(* Logix 5000 AddOnInstructionDefinition export Banner_ZMX_Control; software revision 33.03 *)

TYPE Banner_ZMX_Data :
STRUCT
   Data_In : Banner_ZMX_Data_In;
   Data_Out : Banner_ZMX_Data_Out;
   Unevenness : INT;
END_STRUCT
END_TYPE

TYPE Banner_ZMX_Data_In :
STRUCT
   Input_Ack : INT;
   Reserved1 : INT;
   Sensor_Fault_Code : INT;
   Boot_Count : INT;   // 1 to 65535
   Up_Time : DINT;   // 1 to 4294967295 in ms
   Missed_Trigger_Count : DINT;
   Reserved2 : INT;
   Reserved3 : INT;
   Reserved4 : INT;
   Reserved5 : INT;
   Reserved6 : INT;
   Reserved7 : INT;
   Reserved8 : INT;
   Reserved30 : INT;
   Frame_Number : DINT;
   Invalid_Pixel_Count : DINT;   // 0 to 56576. Pixels with too little light received to be able to measure.
   Saturated_Pixel_Count : DINT;   // 0 to 56576. Pixels with too much light received to be able to measure.
   Conf_Error_Code : INT;
   Reserved9 : INT;
   Fill_Level_Percent : INT;   // 0 to 200
   Peak_Height : INT;   // 0 to 3500 in mm
   Estimated_Item_Count : INT;
   Output_1_PFM : INT;   // 0. 100 to 600 Hz.
   Output_2_PFM : INT;   // 0. 100 to 600 Hz.
   Trigger_Mode : INT;   // 1 = External, 5 = Internal (uses trigger period), 6 = Free run, 10 = Softa
   Trigger_Period : INT;   // 200 to 60000 ms
   Illumination_Power_Percent : INT;   // 1 to 100
   Reserved10 : INT;
   Reserved11 : INT;
   Reserved12 : INT;
   Reserved13 : INT;
   Reserved14 : INT;
   Reserved15 : INT;
   Reserved16 : INT;
   Reserved17 : INT;
   Pitch_Angle : INT;   // -4500 to 4500 (degrees x 100)
   Roll_Angle : INT;   // -4500 to 4500 (degrees x 100)
   Yaw_Angle : INT;   // -18000 to 18000 (degrees x 100)
   Reserved18 : INT;
   Reserved19 : INT;
   Reserved20 : INT;
   Reserved31 : INT;
   Discrete_IO_Polarity : INT;   // 0 = PNP, 1 = NPN, 2 = Push-Pull
   Reserved21 : INT;
   Fill_Level_Limit_Setpoint_Percent : INT;   // 0 to 200 in mm
   Reserved22 : INT;
   Peak_Height_Limit_Setpoint : INT;   // 0 to 2950 mm
   Reserved23 : INT;
   Discrete_Output_1_Control_Mode : INT;   // 0 = Disabled, 1 = Fill % above setpoint, 2 = Peak height aboe setpoint, 9 = Fill % above setpoint or peak height above setpoint, 10 = Pulse Pro 100 to 600 Hz scaled between 0 to 100%, 11 = Pulse Pro 100 to 600 Hz scaled to peak height above bottom of container, 20 = No output, channle used as input.
   Discrete_Output_2_Control_Mode : INT;   // 0 = Disabled, 1 = Fill % above setpoint, 2 = Peak height aboe setpoint, 9 = Fill % above setpoint or peak height above setpoint, 10 = Pulse Pro 100 to 600 Hz scaled between 0 to 100%, 11 = Pulse Pro 100 to 600 Hz scaled to peak height above bottom of container, 20 = No output, channle used as input.
   ROI_Anchor_Point_X : INT;   // -2500 to 2500
   ROI_Anchor_Point_Y : INT;   // -2500 to 2500
   ROI_Anchor_Point_Z : INT;   // 200 to 3000
   ROI_Length_X : INT;   // 50 to 5000
   ROI_Width_Y : INT;   // 50 to 5000
   ROI_Height_Z : INT;   // 50 to 3000
   Reserved24 : INT;
END_STRUCT
END_TYPE

TYPE Banner_ZMX_Data_Out :
STRUCT
   Control_Bits : INT;
   Reserved1 : INT;
   Trigger_Mode : INT;   // 1 = External, 5 = Internal (uses trigger perdio), 6 = Free Run, 10 = Software
   Trigger_Period : INT;   // 100 to 60000 ms
   Illumination_Power_Precent : INT;   // 0 to 100
   Reserved2 : INT;
   Reserved3 : INT;
   Reserved4 : INT;
   Reserved5 : INT;
   Reserved6 : INT;
   Reserved7 : INT;
   Reserved8 : INT;
   Pitch_Angle : INT;   // -4500 to 4500 (degrees x 100)
   Roll_Angle : INT;   // -4500 to 4500 (degrees x 100)
   Yaw_Angle : INT;   // -18000 to 18000 (degrees x 100)
   Reserved9 : INT;
   Reserved10 : INT;
   Reserved11 : INT;
   Discrete_IO_Polarity : INT;   // 0 = PNP, 1 = NPN, 2 = Push Pull
   Reserved12 : INT;
   Fill_Level_Limit_Setpoint_Percent : INT;   // 0 to 200
   Reserved13 : INT;
   Peak_Height_Limit_Setpoint : INT;   // 0 to 2950 in mm
   Reserved14 : INT;
   Discrete_Output_1_Control_Mode : INT;   // 0 = Disabled, 1 = Fill % above setpoint, 2 = Peak height aboe setpoint, 9 = Fill % above setpoint or peak height above setpoint, 10 = Pulse Pro 100 to 600 Hz scaled between 0 to 100%, 11 = Pulse Pro 100 to 600 Hz scaled to peak height above bottom of container, 20 = No output, channle used as input.
   Discrete_Output_2_Control_Mode : INT;   // 0 = Disabled, 1 = Fill % above setpoint, 2 = Peak height aboe setpoint, 9 = Fill % above setpoint or peak height above setpoint, 10 = Pulse Pro 100 to 600 Hz scaled between 0 to 100%, 11 = Pulse Pro 100 to 600 Hz scaled to peak height above bottom of container, 20 = No output, channle used as input.
   ROI_Anchor_Point_X : INT;   // -2500 to 2500 in mm
   ROI_Anchor_Point_Y : INT;   // -2500 to 2500 in mm
   ROI_Anchor_Point_Z : INT;   // 200 to 3000 in mm
   ROI_Length_X : INT;   // 50 to 5000 in mm
   ROI_Width_Y : INT;   // 50 to 5000 in mm
   ROI_Height_Z : INT;   // 50 to 3000 in mm
   Reserved50 : INT[8];
END_STRUCT
END_TYPE

TYPE Banner_ZMX_Full_Recipe :   // Recipe Data elements. for a ZMX unit.
STRUCT
   Trigger_Mode : INT;   // 1 = External, 5 = Internal, 6 = Free Run, 10 = Software
   Trigger_Period : INT;   // 100 to 60000 in ms
   Illumination_Power : INT;   // 0 to 100
   Pitch_Angle : INT;   // -4500 to 4500
   Roll_Angle : INT;   // -4500 to 4500
   Yaw_Angle : INT;   // -18000 to 18000
   Discrete_IO_Polarity : INT;   // 0 = PNP, 1= NPN, 2 = Push Pull
   Fill_Level_Limit_Setpoint_Percent : INT;   // 0 to 200
   Reserved13 : INT;
   Peak_Height_Limit_Setpoint : INT;   // 0 to 2950 in mm
   Reserved14 : INT;
   Discrete_Output_1_Control_Mode : INT;   // 0 = Disabled, 1 = Fill % above setpoint, 2 = Peak height aboe setpoint, 9 = Fill % above setpoint or peak height above setpoint, 10 = Pulse Pro 100 to 600 Hz scaled between 0 to 100%, 11 = Pulse Pro 100 to 600 Hz scaled to peak height above bottom of container, 20 = No output, channle used as input.
   Discrete_Output_2_Control_Mode : INT;   // 0 = Disabled, 1 = Fill % above setpoint, 2 = Peak height aboe setpoint, 9 = Fill % above setpoint or peak height above setpoint, 10 = Pulse Pro 100 to 600 Hz scaled between 0 to 100%, 11 = Pulse Pro 100 to 600 Hz scaled to peak height above bottom of container, 20 = No output, channle used as input.
   ROI_Anchor_X : INT;   // -2500 to 2500 in mm
   ROI_Anchor_Y : INT;   // -2500 to 2500 in mm
   ROI_Anchor_Z : INT;   // 200 to 3000 in mm
   ROI_Length_X : INT;   // 50 to 5000 in mm
   ROI_Length_Y : INT;   // 50 to 5000 in mm
   ROI_Length_Z : INT;   // 50 to 3000 in mm
END_STRUCT
END_TYPE

ADD_ON_INSTRUCTION Banner_ZMX_Control   (* revision 1.2 *)
// Revision note:
// Cyclic operation timing adjusted. Now waits 600 msecs instead of 300 after Cyclic Bit is turned on. Also the error timer is now 5 seconds instead of 3.
VAR_IN_OUT
   BinFill_Update : BOOL; {required}
   Cyclic_Update : BOOL; {required}
   ZMX_Raw_Inputs : INT[68]; {required}
   ZMX_Raw_Outputs : INT[40]; {required}
END_VAR
VAR_INPUT
   ZMX_Status : BOOL; {required}
END_VAR
VAR_IN_OUT
   ZMX : Banner_ZMX_Data; {required}
   Parameter_Update : Banner_ZMX_Full_Recipe; {required}
        .TRIGGER_MODE   // Check Data 1
        .PEAK_HEIGHT_LIMIT_SETPOINT   // Check Data 2
        .DISCRETE_OUTPUT_1_CONTROL_MODE   // Check Data 3
        .DISCRETE_OUTPUT_2_CONTROL_MODE   // Check Data 4
        .ROI_ANCHOR_X   // Check Data 5
        .ROI_ANCHOR_Y   // Check Data 6
        .ROI_ANCHOR_Z   // Check Data 7
        .ROI_LENGTH_X   // Check Data 8
        .ROI_LENGTH_Y   // Check Data 9
        .ROI_LENGTH_Z   // Check Data 10
END_VAR
VAR_OUTPUT
   Busy : BOOL; {visible}
   Done : BOOL; {visible}
   Bin_Error : BOOL; {access Read Only, visible}
   Cyclic_Error : BOOL; {visible}
   Comms_Error : BOOL; {visible}
   Sensor_Fault : INT; {access Read Only, visible}
   Config_Error : INT; {access Read Only, visible}
END_VAR
VAR
   Local : DINT; {access None}
   InData : INT[70]; {access None}
   Timer1 : TIMER := (PRE := 3000); {access None}
   Timer2 : TIMER := (PRE := 5000); {access None}
   Value : DINT[2]; {access None}
END_VAR

ROUTINE Logic   (* ladder *)
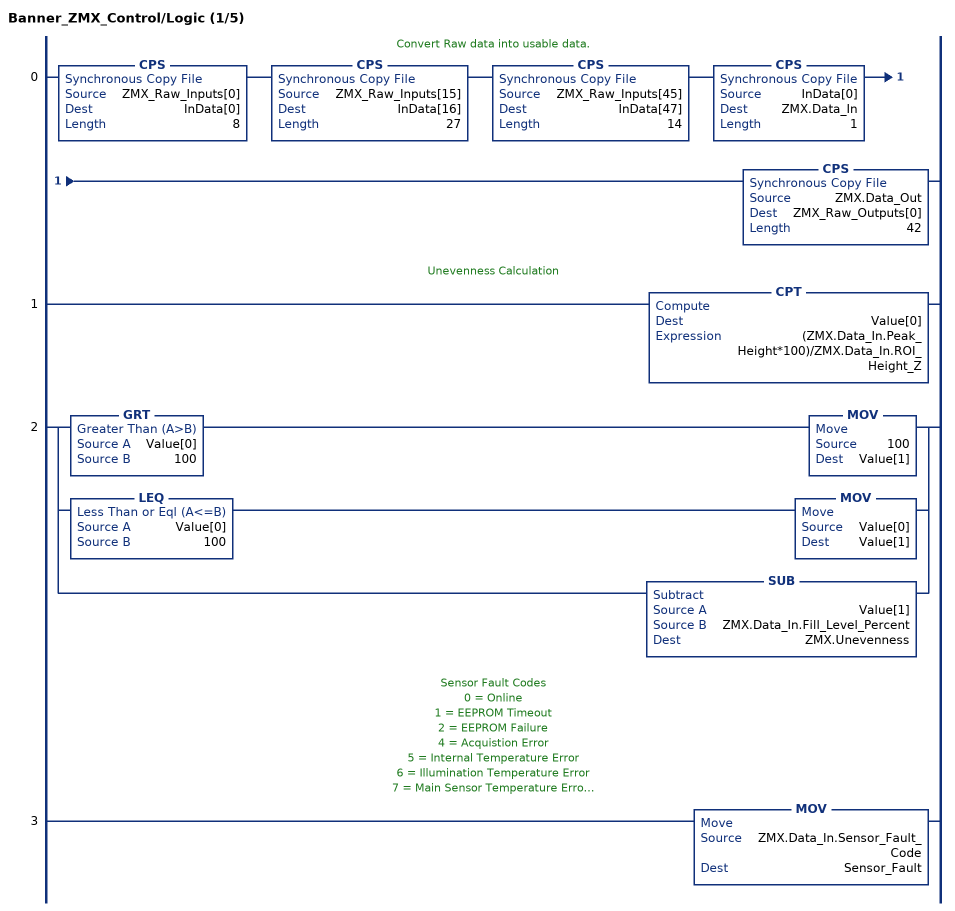
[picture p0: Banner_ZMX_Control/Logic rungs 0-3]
   // Convert Raw data into usable data.
   0: CPS(ZMX_Raw_Inputs[0],InData[0],8)CPS(ZMX_Raw_Inputs[15],InData[16],27)CPS(ZMX_Raw_Inputs[45],InData[47],14)CPS(InData[0],ZMX.Data_In,1)CPS(ZMX.Data_Out,ZMX_Raw_Outputs[0],42);
   // Unevenness Calculation
   1: CPT(Value[0],(ZMX.Data_In.Peak_Height*100)/ZMX.Data_In.ROI_Height_Z);
   2: [GRT(Value[0],100) MOV(100,Value[1]) ,LEQ(Value[0],100) MOV(Value[0],Value[1]) ,SUB(Value[1],ZMX.Data_In.Fill_Level_Percent,ZMX.Unevenness) ];
   // Sensor Fault Codes
   // 0 = Online
   // 1 = EEPROM Timeout
   // 2 = EEPROM Failure
   // 4 = Acquistion Error
   // 5 = Internal Temperature Error
   // 6 = Illumination Temperature Error
   // 7 = Main Sensor Temperature Error
   // 8 = Acquistion Error 2
   // 11 = Laser Operation Error
   // 20 = Internal Test Error
   // 21 = Internal Read Error
   // 22 = Internal Write Error
   // 30 = Laser Power Test Error
   // 31 = Laser Power Read Error
   // 32 = Laser Power Write Error
   // 1000 = Acquistion Error 3
   // 1011 to 1017 = Internal Flash Errors
   // 30000 to 32000 = Boot Loader Error
   3: MOV(ZMX.Data_In.Sensor_Fault_Code,Sensor_Fault);
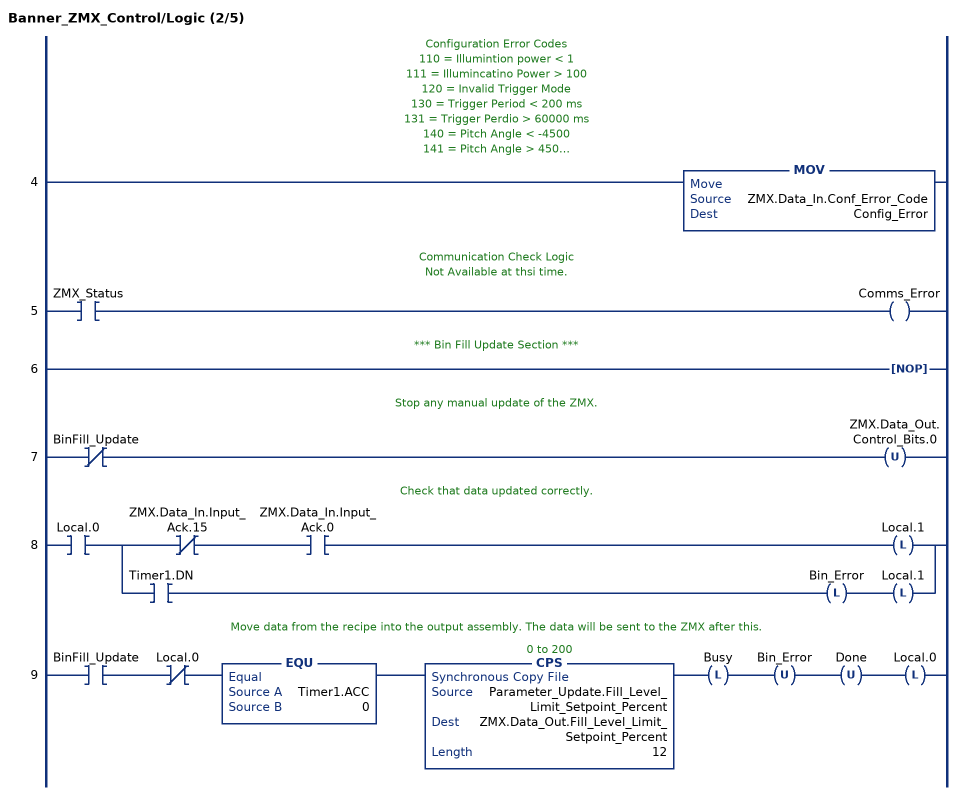
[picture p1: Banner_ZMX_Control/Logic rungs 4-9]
   // Configuration Error Codes
   // 110 = Illumintion power < 1
   // 111 = Illumincatino Power > 100
   // 120 = Invalid Trigger Mode
   // 130 = Trigger Period < 200 ms
   // 131 = Trigger Perdio > 60000 ms
   // 140 = Pitch Angle < -4500
   // 141 = Pitch Angle > 4500
   // 150 = Roll Angle < -4500
   // 151 = Roll Angle > 4500
   // 160 = Yaw Angle < -18000
   // 161 = Yaw Angle > 18000
   // 300 = Invalid Discrete Output
   // 2000 = Anchor Point X < -2500
   // 2001 = Anchor Point X > 2500
   // 2010 = Anchor Point Y < -2500
   // 2011 = Anchor Point Y > 2500
   // 2020 = Anchor Point Z < -2500
   // 2021 = Anchor Point Z > 2500
   // 2030 = Bin Length X < 50
   // 2031 = Bin Length X > 5000
   // 2040 = Bin Width < 50
   // 2041 = Bin Width > 5000
   // 2050 = Bin Width < 50
   // 2051 = Bin Width > 5000
   // 2052 = Invalid Bin Height
   // 2060 = Fill Level Setpoint < 0
   // 2061 = Fill Level Setpoint > 200
   // 2080 = Peak Height Setpoint < 0
   // 2081 = Peak Height Setpoint > Bin Height Z
   // 2100 = Discrete Out 1 Selection Invalid
   // 2110 = Discrete Out 2 Selectino Invalid
   4: MOV(ZMX.Data_In.Conf_Error_Code,Config_Error);
   // Communication Check Logic
   // Not Available at thsi time.
   5: XIC(ZMX_Status)OTE(Comms_Error);
   // *** Bin Fill Update Section ***
   6: NOP();
   // Stop any manual update of the ZMX.
   7: XIO(BinFill_Update)OTU(ZMX.Data_Out.Control_Bits.0);
   // Check that data updated correctly.
   8: XIC(Local.0)[XIO(ZMX.Data_In.Input_Ack.15) XIC(ZMX.Data_In.Input_Ack.0) OTL(Local.1) ,XIC(Timer1.DN) OTL(Bin_Error) OTL(Local.1) ];
   // Move data from the recipe into the output assembly. The data will be sent to the ZMX after this.
   9: XIC(BinFill_Update)XIO(Local.0)EQU(Timer1.ACC,0)CPS(Parameter_Update.Fill_Level_Limit_Setpoint_Percent,ZMX.Data_Out.Fill_Level_Limit_Setpoint_Percent,12)OTL(Busy)OTU(Bin_Error)OTU(Done)OTL(Local.0);
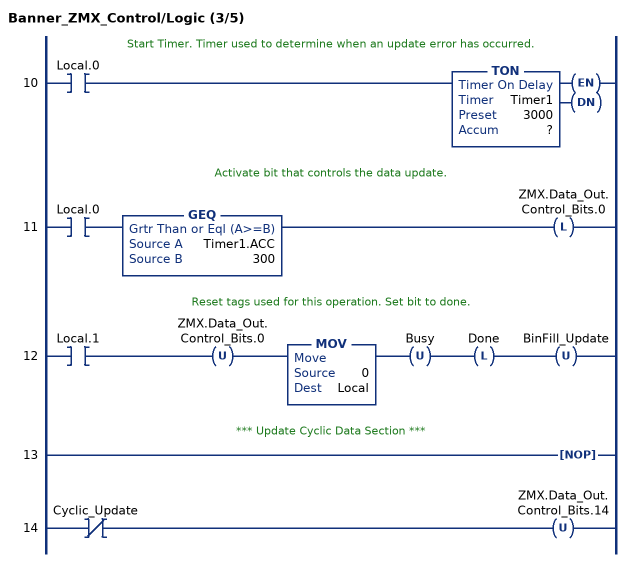
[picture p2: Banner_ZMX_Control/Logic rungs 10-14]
   // Start Timer. Timer used to determine when an update error has occurred.
   10: XIC(Local.0)TON(Timer1,?,?);
   // Activate bit that controls the data update.
   11: XIC(Local.0)GEQ(Timer1.ACC,300)OTL(ZMX.Data_Out.Control_Bits.0);
   // Reset tags used for this operation. Set bit to done.
   12: XIC(Local.1)OTU(ZMX.Data_Out.Control_Bits.0)MOV(0,Local)OTU(Busy)OTL(Done)OTU(BinFill_Update);
   // *** Update Cyclic Data Section ***
   13: NOP();
   14: XIO(Cyclic_Update)OTU(ZMX.Data_Out.Control_Bits.14);
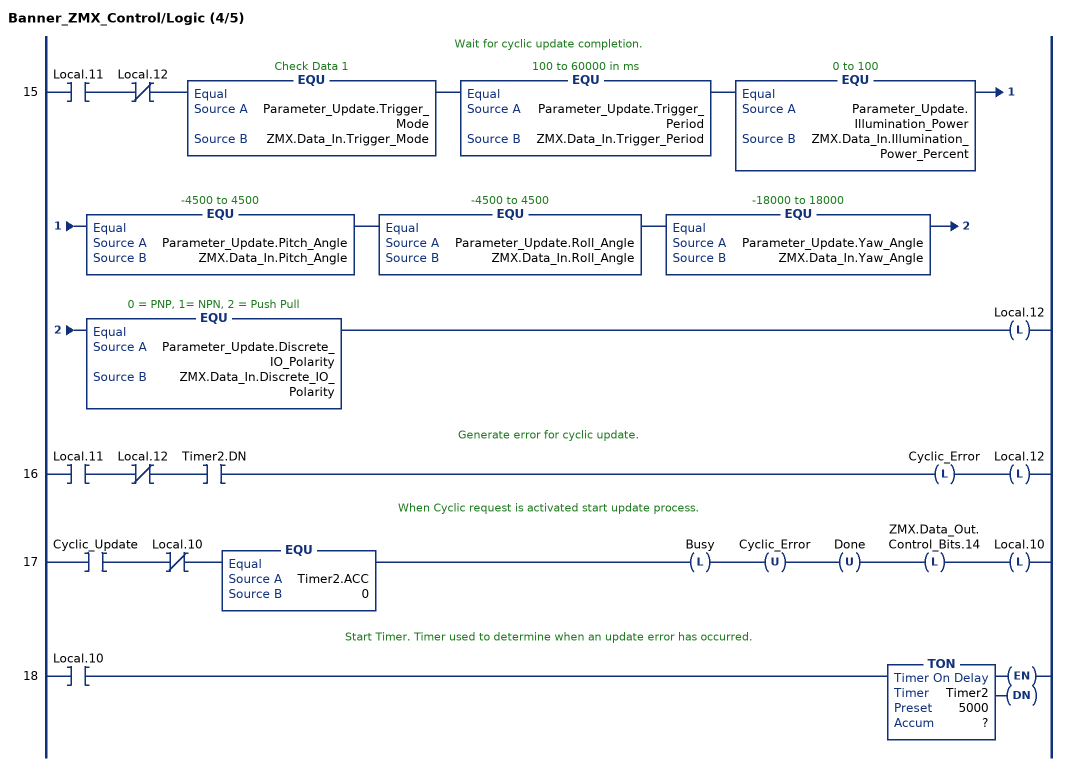
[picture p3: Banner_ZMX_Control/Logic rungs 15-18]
   // Wait for cyclic update completion.
   15: XIC(Local.11)XIO(Local.12)EQU(Parameter_Update.Trigger_Mode,ZMX.Data_In.Trigger_Mode)EQU(Parameter_Update.Trigger_Period,ZMX.Data_In.Trigger_Period)EQU(Parameter_Update.Illumination_Power,ZMX.Data_In.Illumination_Power_Percent)EQU(Parameter_Update.Pitch_Angle,ZMX.Data_In.Pitch_Angle)EQU(Parameter_Update.Roll_Angle,ZMX.Data_In.Roll_Angle)EQU(Parameter_Update.Yaw_Angle,ZMX.Data_In.Yaw_Angle)EQU(Parameter_Update.Discrete_IO_Polarity,ZMX.Data_In.Discrete_IO_Polarity)OTL(Local.12);
   // Generate error for cyclic update.
   16: XIC(Local.11)XIO(Local.12)XIC(Timer2.DN)OTL(Cyclic_Error)OTL(Local.12);
   // When Cyclic request is activated start update process.
   17: XIC(Cyclic_Update)XIO(Local.10)EQU(Timer2.ACC,0)OTL(Busy)OTU(Cyclic_Error)OTU(Done)OTL(ZMX.Data_Out.Control_Bits.14)OTL(Local.10);
   // Start Timer. Timer used to determine when an update error has occurred.
   18: XIC(Local.10)TON(Timer2,?,?);
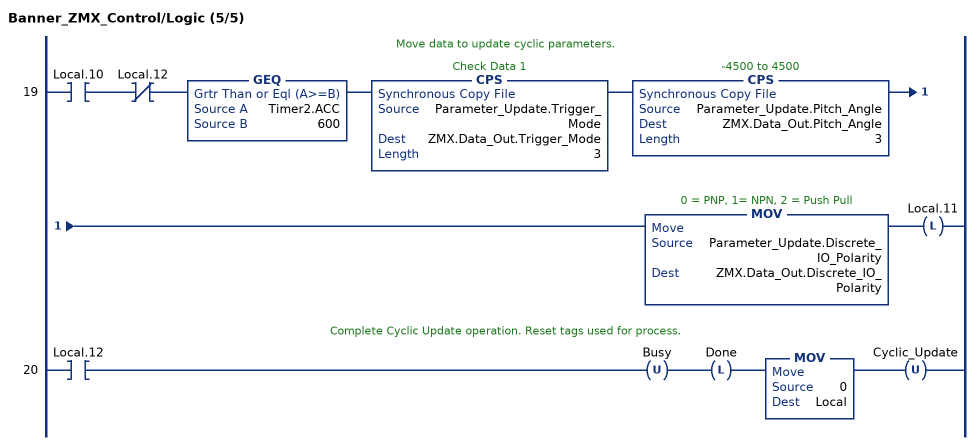
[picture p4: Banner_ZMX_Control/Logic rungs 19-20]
   // Move data to update cyclic parameters.
   19: XIC(Local.10)XIO(Local.12)GEQ(Timer2.ACC,600)CPS(Parameter_Update.Trigger_Mode,ZMX.Data_Out.Trigger_Mode,3)CPS(Parameter_Update.Pitch_Angle,ZMX.Data_Out.Pitch_Angle,3)MOV(Parameter_Update.Discrete_IO_Polarity,ZMX.Data_Out.Discrete_IO_Polarity)OTL(Local.11);
   // Complete Cyclic Update operation. Reset tags used for process.
   20: XIC(Local.12)OTU(Busy)OTL(Done)MOV(0,Local)OTU(Cyclic_Update);
END_ROUTINE
END_ADD_ON_INSTRUCTION
